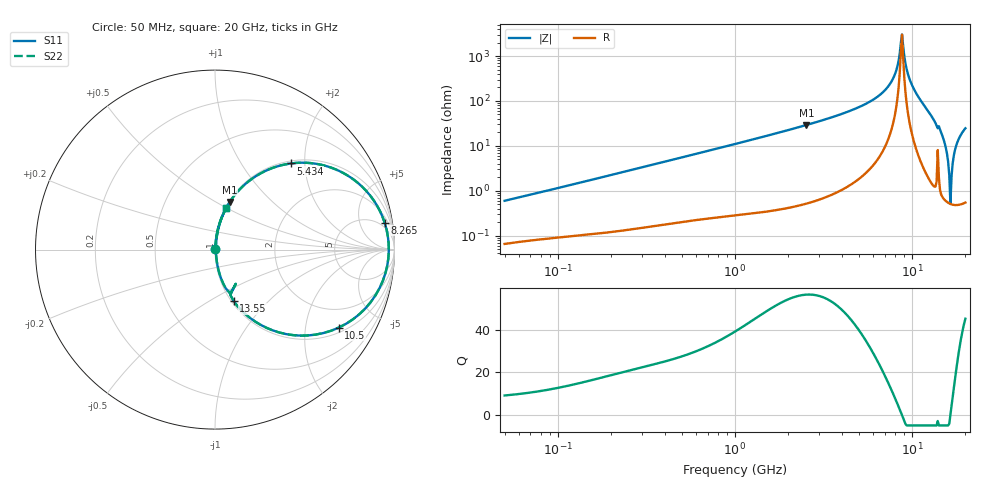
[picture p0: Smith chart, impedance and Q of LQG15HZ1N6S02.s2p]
!Murata Part Number: LQG15HZ1N6S02
!These Parameters are Measured in Series Mode Connection
!  o--[Z]--o
!Port1  Port2
!  o-------o
!Freq. Start=50[MHz] Stop=20[GHz], 401[Steps]
# Hz S RI R 50
!Freq.(Hz) S11(Real) S11(Imag) S21(Real) S21(Imag) S12(Real) S12(Imag) S22(Real) S22(Imag)
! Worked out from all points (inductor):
!   401 points, 50 MHz to 20 GHz, reference 50 ohm
!   read as one part in series: L = 1.86 nH near 51.52 MHz
!   highest Q = 56.6 at 2.531 GHz (marker M1), where L = 1.83 nH
!   self-resonance near 8.645 GHz
!   S11 on the Smith chart (normalised r, x): 50 MHz: 1.00, +0.01; 5.434 GHz: 1.05, +1.70; 8.265 GHz: 3, +12; 10.5 GHz: 1.18, -3.05; 13.55 GHz: 1.02, -0.65; 20 GHz: 1.01, +0.49
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5e7  0.000685 0.00591  0.9993 -0.00591  0.9993 -0.00591  0.000685 0.00591
1.364002e8  0.00125 0.0154  0.9987 -0.0154  0.9987 -0.0154  0.00125 0.0154
3.721004e8  0.00337 0.041  0.9966 -0.041  0.9966 -0.041  0.00337 0.041
1e9  0.0146 0.1077  0.9854 -0.1077  0.9854 -0.1077  0.0146 0.1077
2.531158e9  0.0821 0.2658  0.9179 -0.2658  0.9179 -0.2658  0.0821 0.2658
2.728004e9  0.0955 0.2852  0.9045 -0.2852  0.9045 -0.2852  0.0955 0.2852
5.433528e9  0.4207 0.4798  0.5793 -0.4798  0.5793 -0.4798  0.4207 0.4798
7.442007e9  0.8226 0.3477  0.1774 -0.3477  0.1774 -0.3477  0.8226 0.3477
8.264682e9  0.945 0.151  0.055 -0.151  0.055 -0.151  0.945 0.151
8.774992e9  0.9685 -0.0049  0.0315 0.0049  0.0315 0.0049  0.9685 -0.0049
9.600142e9  0.8941 -0.2549  0.1059 0.2549  0.1059 0.2549  0.8941 -0.2549
1.050288e10  0.69 -0.4344  0.31 0.4344  0.31 0.4344  0.69 -0.4344
1.183995e10  0.3588 -0.462  0.6412 0.462  0.6412 0.462  0.3588 -0.462
1.354865e10  0.1036 -0.2862  0.8964 0.2862  0.8964 0.2862  0.1036 -0.2862
1.504638e10  0.0257 -0.1362  0.9743 0.1362  0.9743 0.1362  0.0257 -0.1362
1.573793e10  0.00997 -0.0659  0.99 0.0659  0.99 0.0659  0.00997 -0.0659
1.597544e10  0.00727 -0.0435  0.9927 0.0435  0.9927 0.0435  0.00727 -0.0435
1.646126e10  0.00504 -0.000339  0.995 0.000339  0.995 0.000339  0.00504 -0.000339
1.696185e10  0.00652 0.0408  0.9935 -0.0408  0.9935 -0.0408  0.00652 0.0408
1.747767e10  0.0112 0.0798  0.9888 -0.0798  0.9888 -0.0798  0.0112 0.0798
1.800918e10  0.0186 0.1166  0.9814 -0.1166  0.9814 -0.1166  0.0186 0.1166
2e10  0.0615 0.2294  0.9385 -0.2294  0.9385 -0.2294  0.0615 0.2294
